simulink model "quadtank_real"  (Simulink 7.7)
settings: Solver=ode45  StartTime=0.0  StopTime=150  RelTol=1e-6
PreLoadFcn:
  | init_quadtank
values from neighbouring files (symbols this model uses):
  Aaw = tf([1 2 1],[1])    [init_quadtank.m]
  C1 = 1/(s+1)    [init_quadtank.m]
  C2 = 1/(s+1)    [init_quadtank.m]
  W1 = eye(2)    [init_quadtank.m]
  W2 = eye(2)    [init_quadtank.m]
libraries: cstblocks x4

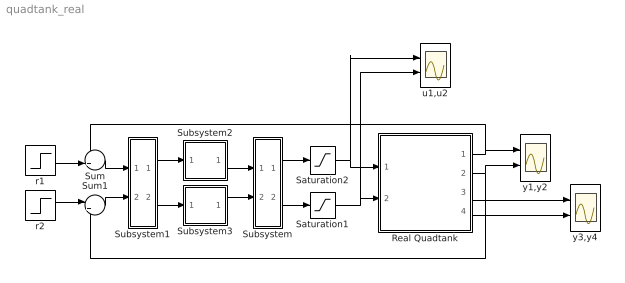
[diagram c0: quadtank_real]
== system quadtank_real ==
  Real Quadtank : Subsystem  AncestorBlock=tank/Real Quadtank  mask{h=0.05}
  Saturation1 : Saturate  UpperLimit=10  LowerLimit=0
  Saturation2 : Saturate  UpperLimit=10  LowerLimit=0
  Subsystem : Subsystem
  Subsystem1 : Subsystem
  Subsystem2 : Subsystem  mask(Controller C1){aw=off}
      mask prompts: aw "Antiwindup"
      mask help: Uses the LTI variable C1 from the workspace
  Subsystem3 : Subsystem  mask(Controller C2){aw=off}
      mask prompts: aw "Antiwindup"
      mask help: Uses the LTI variable C2 from the workspace
  Sum : Sum  Inputs=-+|
  Sum1 : Sum  Inputs=|+-
  r1 : Step  Time=50  Before=5  After=6  SampleTime=0
  r2 : Step  Time=100  Before=5  After=6  SampleTime=0
  u1,u2 : Scope  NumInputPorts=2
  y1,y2 : Scope  NumInputPorts=2
  y3,y4 : Scope  NumInputPorts=2
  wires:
  Real Quadtank/1(y1) -> Sum/1, y1,y2/1
  Real Quadtank/2(y2) -> Sum1/2, y1,y2/2
  r2/1 -> Sum1/1
  Real Quadtank/3(y3) -> y3,y4/1
  Real Quadtank/4(y4) -> y3,y4/2
  Saturation2/1 -> u1,u2/1, Real Quadtank/1(u1)
  Saturation1/1 -> u1,u2/2, Real Quadtank/2(u2)
  Subsystem2/1(u) -> Subsystem/1(In1)
  Subsystem3/1(u) -> Subsystem/2(In2)
  Subsystem1/1(Out1) -> Subsystem2/1(e)
  Subsystem1/2(Out2) -> Subsystem3/1(e)
  Subsystem/1(Out1) -> Saturation2/1
  Subsystem/2(Out2) -> Saturation1/1
  Sum/1 -> Subsystem1/1(In1)
  Sum1/1 -> Subsystem1/2(In2)
  r1/1 -> Sum/2

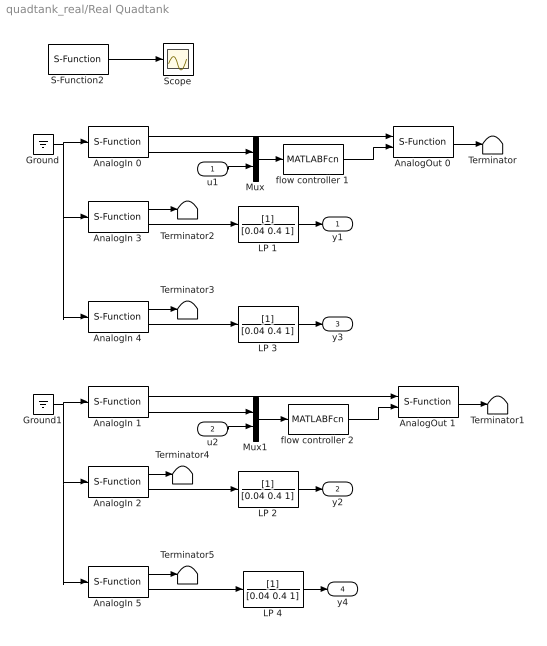
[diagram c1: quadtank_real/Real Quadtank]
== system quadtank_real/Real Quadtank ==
  u1 : Inport
  u2 : Inport  Port=2
  AnalogIn 0 : S-Function  FunctionName=analogin  Parameters=h [35]  EnableBusSupport=off
  AnalogIn 1 : S-Function  FunctionName=analogin  Parameters=h [34]  EnableBusSupport=off
  AnalogIn 2 : S-Function  FunctionName=analogin  Parameters=h [33]  EnableBusSupport=off
  AnalogIn 3 : S-Function  FunctionName=analogin  Parameters=h [31]  EnableBusSupport=off
  AnalogIn 4 : S-Function  FunctionName=analogin  Parameters=h [30]  EnableBusSupport=off
  AnalogIn 5 : S-Function  FunctionName=analogin  Parameters=h [32]  EnableBusSupport=off
  AnalogOut 0 : S-Function  FunctionName=analogout  Parameters=h [31]  EnableBusSupport=off
  AnalogOut 1 : S-Function  FunctionName=analogout  Parameters=h [30]  EnableBusSupport=off
  Ground : Ground
  Ground1 : Ground
  LP {1..4} (4 alike) : TransferFcn  Denominator=[0.04 0.4 1]
  Mux : Mux  Inputs=2
  Mux1 : Mux  Inputs=2
  S-Function2 : S-Function  FunctionName=realtimer  Parameters=h  EnableBusSupport=off
  Scope : Scope
  Terminator{,1..5} (6 alike) : Terminator
  flow controller 1 : MATLABFcn  MATLABFcn=flowCtrl1  SampleTime=0.01
  flow controller 2 : MATLABFcn  MATLABFcn=flowCtrl2  SampleTime=0.01
  y1 : Outport
  y2 : Outport  Port=2
  y3 : Outport  Port=3
  y4 : Outport  Port=4
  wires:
  S-Function2/1 -> Scope/1
  AnalogIn 0/1 -> AnalogOut 0/1
  AnalogOut 0/1 -> Terminator/1
  AnalogIn 1/1 -> AnalogOut 1/1
  AnalogOut 1/1 -> Terminator1/1
  AnalogIn 3/2 -> LP 1/1
  AnalogIn 4/2 -> LP 3/1
  Ground/1 -> AnalogIn 0/1, AnalogIn 3/1, AnalogIn 4/1
  AnalogIn 3/1 -> Terminator2/1
  AnalogIn 4/1 -> Terminator3/1
  AnalogIn 2/2 -> LP 2/1
  AnalogIn 5/2 -> LP 4/1
  Ground1/1 -> AnalogIn 5/1, AnalogIn 2/1, AnalogIn 1/1
  AnalogIn 2/1 -> Terminator4/1
  AnalogIn 5/1 -> Terminator5/1
  u1/1 -> Mux/2
  Mux/1 -> flow controller 1/1
  flow controller 1/1 -> AnalogOut 0/2
  u2/1 -> Mux1/2
  Mux1/1 -> flow controller 2/1
  flow controller 2/1 -> AnalogOut 1/2
  AnalogIn 1/2 -> Mux1/1
  AnalogIn 0/2 -> Mux/1
  LP 1/1 -> y1/1
  LP 3/1 -> y3/1
  LP 2/1 -> y2/1
  LP 4/1 -> y4/1

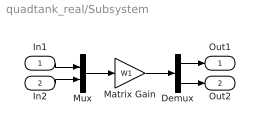
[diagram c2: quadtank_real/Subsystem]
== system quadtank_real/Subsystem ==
  In1 : Inport
  In2 : Inport  Port=2
  Demux : Demux  Outputs=2
  Matrix Gain : Gain  Gain=W1  Multiplication=Matrix(K*u)
  Mux : Mux  Inputs=2
  Out1 : Outport
  Out2 : Outport  Port=2
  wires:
  Demux/1 -> Out1/1
  In1/1 -> Mux/1
  Demux/2 -> Out2/1
  In2/1 -> Mux/2
  Mux/1 -> Matrix Gain/1
  Matrix Gain/1 -> Demux/1

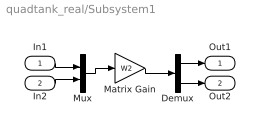
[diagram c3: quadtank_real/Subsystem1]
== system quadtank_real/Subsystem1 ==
  In1 : Inport
  In2 : Inport  Port=2
  Demux : Demux  Outputs=2
  Matrix Gain : Gain  Gain=W2  Multiplication=Matrix(K*u)
  Mux : Mux  Inputs=2
  Out1 : Outport
  Out2 : Outport  Port=2
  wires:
  Matrix Gain/1 -> Demux/1
  Mux/1 -> Matrix Gain/1
  In2/1 -> Mux/2
  Demux/2 -> Out2/1
  In1/1 -> Mux/1
  Demux/1 -> Out1/1

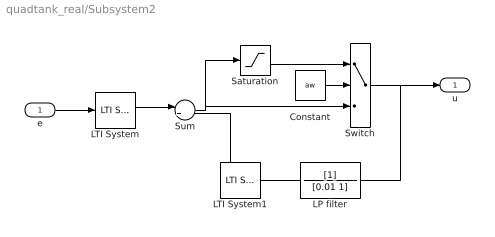
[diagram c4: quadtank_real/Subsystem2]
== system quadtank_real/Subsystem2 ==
  e : Inport
  Constant : Constant  Value=aw
  LP filter : TransferFcn  Denominator=[0.01 1]
  LTI System : cstblocks/LTI System  SystemSampleTime=-1  sys=tf(C1.num{:},1)/Aaw  IC=[]
  LTI System1 : cstblocks/LTI System  SystemSampleTime=-1  sys=(Aaw-tf(C1.den{:},1))/Aaw  IC=[]
  Saturation : Saturate  UpperLimit=10  LowerLimit=0
  Sum : Sum  Inputs=|++
  Switch : Switch  Threshold=0.5
  u : Outport
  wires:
  LP filter/1 -> LTI System1/1
  Sum/1 -> Saturation/1, Switch/3
  Saturation/1 -> Switch/1
  Switch/1 -> LP filter/1, u/1
  Constant/1 -> Switch/2
  LTI System1/1 -> Sum/2
  LTI System/1 -> Sum/1
  e/1 -> LTI System/1

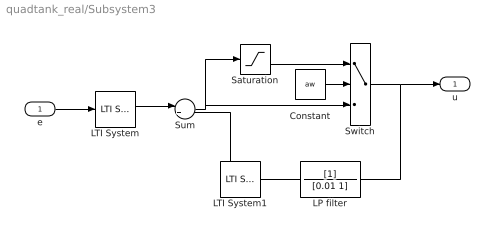
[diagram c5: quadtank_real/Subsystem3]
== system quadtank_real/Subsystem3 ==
  e : Inport
  Constant : Constant  Value=aw
  LP filter : TransferFcn  Denominator=[0.01 1]
  LTI System : cstblocks/LTI System  SystemSampleTime=-1  sys=tf(C2.num{:},1)/Aaw  IC=[]
  LTI System1 : cstblocks/LTI System  SystemSampleTime=-1  sys=(Aaw-tf(C2.den{:},1))/Aaw  IC=[]
  Saturation : Saturate  UpperLimit=10  LowerLimit=0
  Sum : Sum  Inputs=|++
  Switch : Switch  Threshold=0.5
  u : Outport
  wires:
  e/1 -> LTI System/1
  LTI System/1 -> Sum/1
  LTI System1/1 -> Sum/2
  Constant/1 -> Switch/2
  Switch/1 -> u/1, LP filter/1
  Saturation/1 -> Switch/1
  Sum/1 -> Switch/3, Saturation/1
  LP filter/1 -> LTI System1/1
